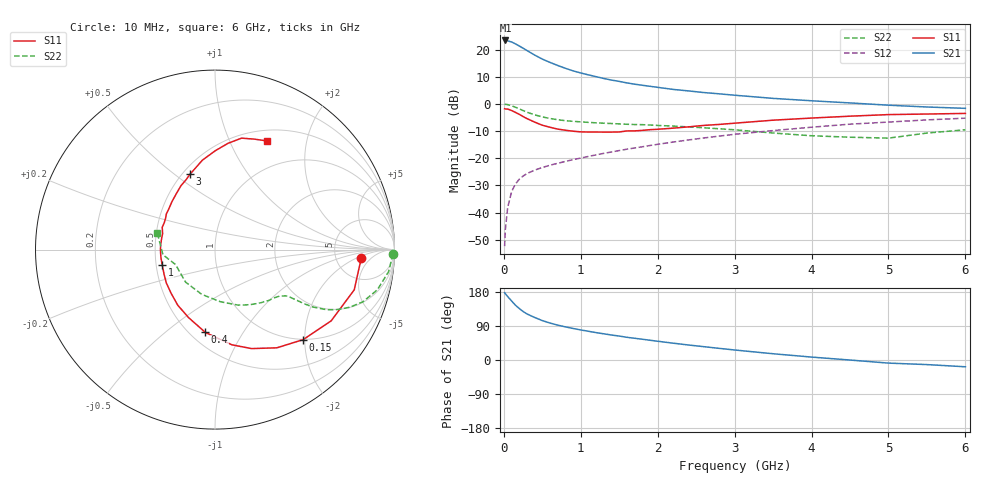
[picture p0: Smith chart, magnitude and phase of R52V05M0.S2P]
! SIEMENS Small Signal Semiconductors
! BFR183
! Si NPN RF Bipolar Junction Transistor in SOT23
! VCE = 2 V  IC = 5 mA
! Common Emitter S-Parameters:  May  1996
# GHz  S  MA  R  50
!  f  S11  S21  S12  S22
! GHz  MAG  ANG  MAG  ANG  MAG  ANG  MAG  ANG
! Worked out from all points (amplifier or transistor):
!   36 points, 10 MHz to 6 GHz, reference 50 ohm
!   highest |S21| = 23.4 dB at 20 MHz (marker M1)
!   |S21| within 3 dB of that: start of sweep to 259 MHz
!   unconditionally stable (mu >= 1): 1.002 GHz to 2.653 GHz
!   at 250 MHz: K = 0.42, MSG = 23.6 dB, |S12| = -26.6 dB
!   at 1.4 GHz: K = 1.07, MAG = 11.7 dB, |S12| = -17.7 dB
!   at 6 GHz: K = 0.89, MSG = 1.8 dB, |S12| = -5.2 dB
!   lowest NFmin = 1.15 dB at 450 MHz
!   S11 on the Smith chart (normalised r, x): 10 MHz: 9.15, -2.67; 150 MHz: 0.99, -1.97; 400 MHz: 0.59, -0.70; 1 GHz: 0.54, -0.10; 3 GHz: 0.55, +0.57; 6 GHz: 0.63, +1.39
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0.01  0.8172 -3.4  14.79 177.6  0.0024 88.5  0.9898 -1.4
0.02  0.8102 -6.6  14.83 174.8  0.0049 84.5  0.986 -3.0
0.05  0.8076 -16.1  14.58 167.5  0.0124 81.2  0.9747 -7.3
0.1  0.7593 -31.5  13.91 155.9  0.024 74.8  0.9318 -13.9
0.15  0.7021 -45.6  12.84 144.7  0.0335 67.7  0.8731 -19.5
0.2  0.6466 -57.8  11.75 136.0  0.041 63.8  0.8158 -23.2
0.25  0.5881 -69.7  10.69 128.0  0.047 60.1  0.7571 -26.2
0.3  0.5389 -79.9  9.689 121.6  0.0522 58.0  0.7066 -28.3
0.4  0.4643 -96.7  7.991 112.3  0.0604 55.7  0.6319 -30.4
0.5  0.4063 -111.3  6.725 104.0  0.0676 54.6  0.5788 -31.3
0.6  0.3729 -123.8  5.845 97.5  0.0745 54.7  0.5407 -31.7
0.7  0.3447 -135.3  5.133 92.1  0.0807 55.4  0.5137 -32.1
0.8  0.3286 -145.7  4.55 87.4  0.0875 55.6  0.4929 -32.4
1  0.3065 -163.4  3.73 79.3  0.1009 56.7  0.4688 -33.3
1.1  0.3045 -171.9  3.441 75.8  0.1082 57.2  0.4588 -34.3
1.6  0.3191 157.2  2.451 59.9  0.147 58.1  0.4234 -39.4
2.2  0.3591 131.9  1.859 44.4  0.1991 56.2  0.3923 -48.9
3  0.4434 108.1  1.452 26.4  0.2766 49.8  0.3347 -67.5
3.5  0.5034 98.0  1.27 16.5  0.3238 44.3  0.292 -84.1
4.5  0.5967 83.0  1.047 -0.1  0.4253 32.2  0.2444 -132.1
5.5  0.6536 70.3  0.881 -12.1  0.5097 19.5  0.2915 -174.3
6  0.6709 64.5  0.832 -17.9  0.5485 11.4  0.3353 163.7
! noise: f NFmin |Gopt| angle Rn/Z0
0.45  1.15  0.25  40  0.26
0.9  1.2  0.25  93  0.22
1.8  1.95  0.32  170  0.13
